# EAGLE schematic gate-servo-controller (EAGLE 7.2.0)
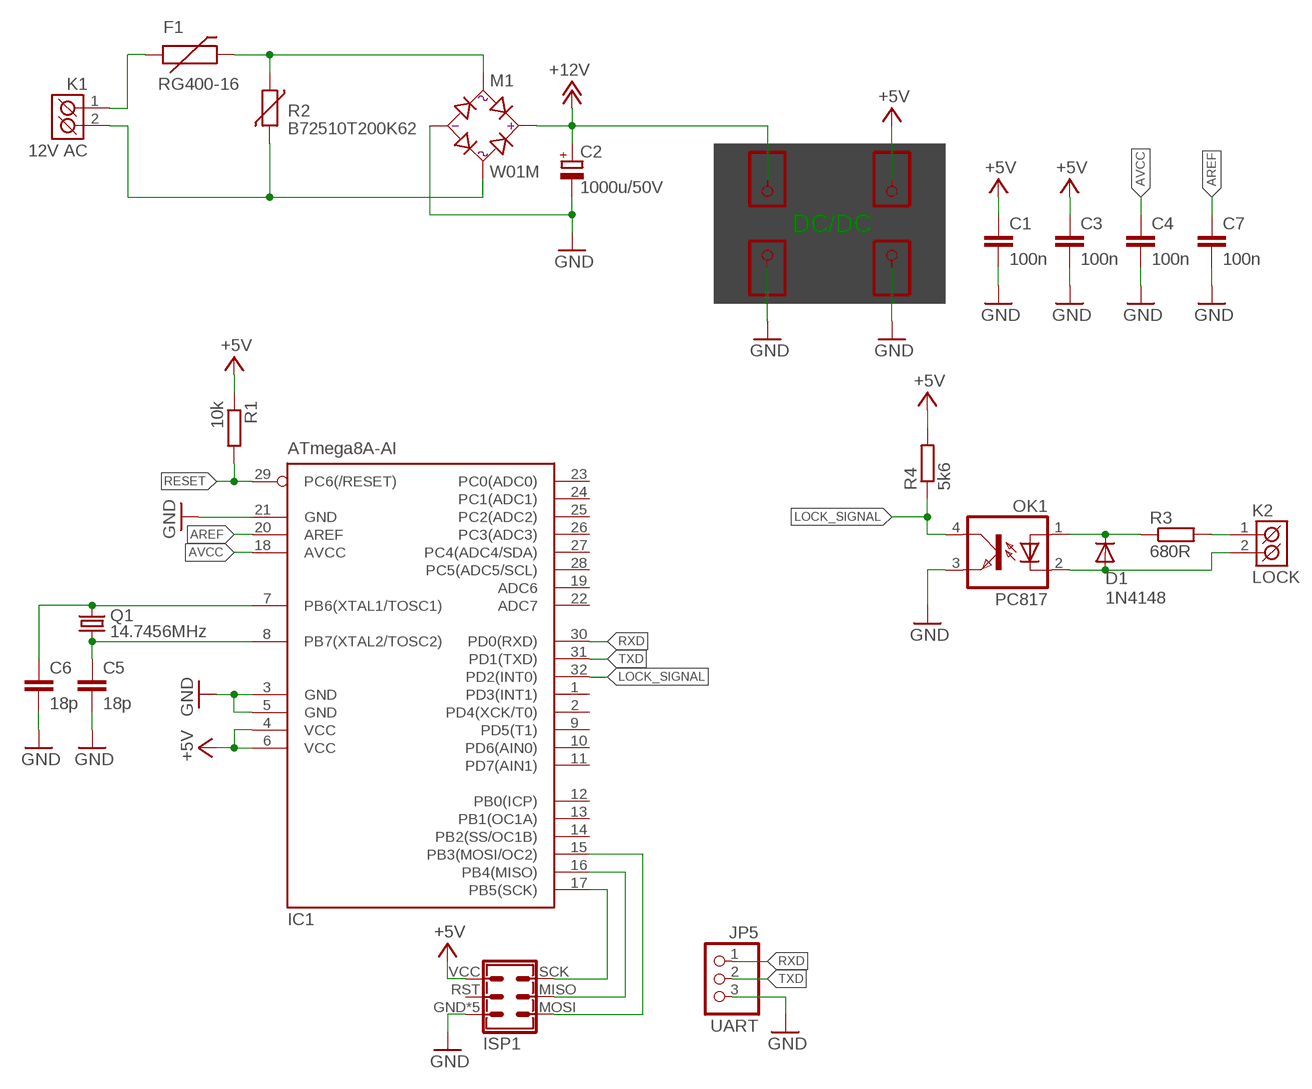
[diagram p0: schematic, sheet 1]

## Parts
C1  100n  C-EUC0805K  [C0805K]
C2  1000u/50V  CPOL-EUE5-13  [E5-13]
C3  100n  C-EUC0805K  [C0805K]
C4  100n  C-EUC0805K  [C0805K]
C5  18p  C-EUC0805K  [C0805K]
C6  18p  C-EUC0805K  [C0805K]
C7  100n  C-EUC0805K  [C0805K]
D1  1N4148  DIODE-MINIMELF  [MINIMELF]
F1  RG400-16  PTCPTH  [PTC]
IC1  ATmega8A-AI  MEGA8-AI  [TQFP32-08]
ISP1  MLW10-0  [MLW10G]
JP1  12V  PINHD-1X1  [1X01]
JP2  5V  PINHD-1X1  [1X01]
JP3  GND  PINHD-1X1  [1X01]
JP4  GND  PINHD-1X1  [1X01]
JP5  UART  PINHD-1X3  [1X03]
K1  12V AC  ARK500/2  [ARK500/2]
K2  LOCK  ARK500/2  [ARK500/2]
M1  W01M  D-B250C1500_MUSTEK  [DM_WOM]
OK1  PC817  [DIL04]
Q1  14.7456MHz  CRYSTALHC49U-V  [HC49U-V]
R1  10k  R-EU_R0805  [R0805]
R2  B72510T200K62  VARISTORCN0805  [CT/CN0805]
R3  680R  R-EU_R0805  [R0805]
R4  5k6  R-EU_R0805  [R0805]

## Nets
+5V: C1.1 C3.1 IC1.4(VCC) IC1.6(VCC) ISP1.VCC JP2.1 R1.1 R4.2
+12V: C2.+ JP1.1 M1.+
AREF: C7.1 IC1.20(AREF)
AVCC: C4.1 IC1.18(AVCC)
GND: C1.2 C2.- C3.2 C4.2 C5.2 C6.2 C7.2 IC1.3(GND) IC1.5(GND) IC1.21(GND) ISP1.GND ISP1.GND@1(GND) ISP1.GND@2(GND) ISP1.GND@3(GND) ISP1.GND@4(GND) JP3.1 JP4.1 JP5.3 M1.- OK1.3(EMIT)
LOCK_SIGNAL: IC1.32(PD2(INT0)) OK1.4(COL) R4.1
N$1: C6.1 IC1.7(PB6(XTAL1/TOSC1)) Q1.2
N$2: F1.P$1 K1.1(K1)
N$3: K1.2(K2) M1.AC2 R2.2
N$4: C5.1 IC1.8(PB7(XTAL2/TOSC2)) Q1.1
N$5: IC1.17(PB5(SCK)) ISP1.SCK
N$6: IC1.16(PB4(MISO)) ISP1.MISO
N$7: F1.P$2 M1.AC1 R2.1
N$8: IC1.15(PB3(MOSI/OC2)) ISP1.MOSI
N$9: D1.C OK1.1(A) R3.1
N$10: K2.1(K1) R3.2
N$11: D1.A K2.2(K2) OK1.2(C)
RESET: IC1.29(PC6(/RESET)) R1.2
RXD: IC1.30(PD0(RXD)) JP5.1
TXD: IC1.31(PD1(TXD)) JP5.2
Unconnected: IC1.1(PD3(INT1)) IC1.2(PD4(XCK/T0)) IC1.9(PD5(T1)) IC1.10(PD6(AIN0)) IC1.11(PD7(AIN1)) IC1.12(PB0(ICP)) IC1.13(PB1(OC1A)) IC1.14(PB2(SS/OC1B)) IC1.19(ADC6) IC1.22(ADC7) IC1.23(PC0(ADC0)) IC1.24(PC1(ADC1)) IC1.25(PC2(ADC2)) IC1.26(PC3(ADC3)) IC1.27(PC4(ADC4/SDA)) IC1.28(PC5(ADC5/SCL)) ISP1.RST

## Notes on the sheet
- DC/DC

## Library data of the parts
C1 C3-C7 = rcl:C-EU: CAPACITOR, European symbol
C2 = rcl:CPOL-EU: POLARIZED CAPACITOR, European symbol
D1 = diode:DIODE-: DIODE
F1 = SparkFun-PowerIC:PTC: Resettable Fuse PTC
IC1 = atmel:MEGA8: MICROCONTROLLER 8 Kbytes FLASH, 1 kbytes SRAM, 512 bytes EEPROM, USART, 6-channel 10 bit ADC, 2-channel 8 bit ADC Pin compatible with Atmega48, ATMega88, ATMega168 Source: avr.lbr; MPN: ATMEGA8-16AU; OC_FARNELL: 9171371; OC_NEWARK: 73M8863
ISP1 = ##MJ:MLW10: Programovací konektor (10-pin)
JP1-JP4 = pinhead:PINHD-1X1: PIN HEADER
JP5 = pinhead:PINHD-1X3: PIN HEADER
K1 K2 = #PaJa_konektory:ARK500/2: Svorkovnice - roztec 5mm - dvojita
M1 = #PaJa_31:D-?_MUSTEK: Diodovy mustek - Graetz
OK1 = optocoupler:PC817: SHARP OPTO COUPLER; MPN: PC817X4J000F; OC_FARNELL: 9707727; OC_NEWARK: 97K7059
Q1 = crystal:CRYSTAL: CRYSTAL; OC_FARNELL: 1666969; OC_NEWARK: unknown
R1 R3 R4 = rcl:R-EU_: RESISTOR, European symbol
R2 = varistor:VARISTOR: VARISTOR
